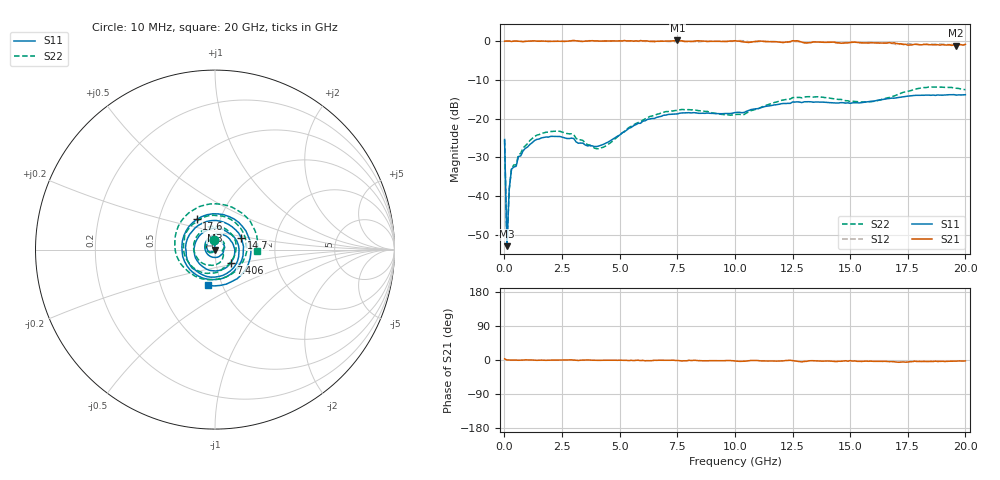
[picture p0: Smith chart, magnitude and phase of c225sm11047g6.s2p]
! 7/29/2020 12:35:05 PM
! D:\C225SM11047G6.S2P
! CHANNEL.1
! TR.MEASUREMENT
! CORRECTED.DATA
# GHZ S RI R 50.0
! FREQ.GHZ  S11RE  S11IM  S21RE  S21IM  S12RE  S12IM  S22RE  S22IM
!; PortSelection: Port_12
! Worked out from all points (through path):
!   201 points, 10 MHz to 20 GHz, reference 50 ohm
!   highest |S21| = 0.16 dB at 7.506 GHz (marker M1); lowest = -1.2 dB at 19.6 GHz (marker M2)
!   lowest |S11| = -52.9 dB at 110 MHz (marker M3), VSWR 1.00, Z = 50 - j0.222 ohm
!   |S11| at or under -10 dB: start of sweep to end of sweep
!   |S22| runs from -52.9 to -11.8 dB; largest |S21 - S12| = 0.052
!   S11 on the Smith chart (normalised r, x): 10 MHz: 0.99, +0.11; 7.406 GHz: 1.18, -0.17; 14.7 GHz: 1.33, +0.18; 17.6 GHz: 0.77, +0.27; 20 GHz: 0.86, -0.36
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0.01  -0.00368 0.0536  0.995 0.0542  0.9945 0.0527  -0.00336 0.0532
0.10995  -0.000467 -0.00222  0.9998 0.00354  1 0.00236  -0.000791 -0.00213
0.2099  -0.00477 -0.0114  1 -0.00184  1 -0.00198  -0.00373 -0.0115
0.30985  -0.0199 -0.0102  0.9879 -0.00457  0.9902 -0.00304  -0.0196 -0.0119
0.8096  -0.0376 -0.00739  0.9817 -0.00191  0.9864 -0.00554  -0.0406 -0.0103
2.009  -0.0113 0.058  0.9907 -0.00663  0.9927 -0.00648  -0.0179 0.0658
3.4083  0.0429 -0.0223  0.9882 -0.00334  0.9912 -0.00101  0.0509 0.0118
4.10795  -0.0146 -0.0421  1.001 -0.0158  0.9957 -0.00467  0.0404 -0.00591
6.70665  0.102 0.027  0.993 -0.0105  0.9962 -0.0304  -0.1144 -0.0146
7.4063  0.0889 -0.0729  1.009 -0.0187  0.9836 -0.0318  -0.0802 0.0989
7.50625  0.0789 -0.0838  1.018 -0.022  0.9788 -0.0208  -0.0669 0.1084
8.90555  -0.1134 -0.0296  0.9899 -0.0309  0.9949 -0.0293  0.1165 0.0337
10.005  0.000982 0.1198  1.01 -0.0448  1.001 -0.0237  0.0772 -0.0825
12.004  -0.0236 -0.1536  0.9596 -0.0456  0.9635 -0.0508  -0.168 -0.0343
13.4033  -0.1268 0.1021  0.9722 -0.0326  0.976 -0.0317  0.0134 0.1892
14.70265  0.1455 0.0672  0.9422 -0.0448  0.936 -0.0269  0.1711 -0.0314
15.8021  0.0388 -0.1611  0.9398 -0.056  0.9565 -0.0561  0.03 -0.1625
16.70165  -0.17 -0.0648  0.9536 -0.0719  0.935 -0.0841  -0.1289 -0.1358
17.6012  -0.1014 0.1683  0.8889 -0.068  0.9196 -0.0751  -0.2238 0.0466
18.8006  0.1964 0.0464  0.8958 -0.0606  0.9065 -0.0452  0.0341 0.2527
19.6002  0.0916 -0.179  0.8748 -0.0452  0.9071 -0.0285  0.2222 0.1073
20  -0.0376 -0.1999  0.9063 -0.0368  0.901 -0.0361  0.2359 -0.00777
